(* FB_CylinderDiag	- number of control signals控制信号数量:
							one direction is controllable一个方向是可控的
					- type of feedback signal反馈信号的类型:
							feedback in base and work position基准和工作位置的反馈
					- with position diagnosis带位置诊断				*)
					
FUNCTION_BLOCK FB_CylinderDiag EXTENDS FB_Cylinder
VAR_INPUT
	tTimeOut 	 		: TIME;						// Time for watchdog that monitores if cylinder reaches base/work position监视气缸是否到达基准/工作位置的看门狗的时间
END_VAR
VAR_OUTPUT
	bError				: BOOL;						// Error signal (diagnosed from position watchdog)错误信号（由位置看门狗诊断）
	sErrorMsg			: STRING;					// Error message错误消息
END_VAR
VAR
	fbTriggerError		: R_TRIG;					// Trigger to recognize rising edge of error识别错误上升沿的触发器
	bErrorMove			: BOOL;						// Move error移动错误
	fbTimerWatchDog		: TON;						// Watchdog timer for monitoring if cylinder reaches base/work position看门狗计时器，用于监测气缸是否到达基准/工作位置
END_VAR

// =========================================================
;
// =========================================================

METHOD PROTECTED Diag
VAR_INPUT
END_VAR
// =========================================================
// Timer starts when cylinder is not in base and work position当气缸不在基准和工作位置时，计时器启动
	
	IF NOT bAtBasePos AND NOT bAtWorkPos THEN
		fbTimerWatchDog(IN := TRUE,
						PT := tTimeOut);
	ELSE
		fbTimerWatchDog(IN := FALSE,
						PT := tTimeOut);
	END_IF

// =========================================================
// Error if cylinder does not reach base or work position气缸未到达基准或工作位置时报错
	
	fbTriggerError(CLK := fbTimerWatchDog.Q);
	
	bError := fbTimerWatchDog.Q;
	
	IF fbTriggerError.Q THEN
		bErrorMove := bMoveToWork;
	END_IF
	
	IF bError THEN
		IF bErrorMove = bMoveToWork THEN
			IF bMoveToWork THEN
				sErrorMsg := 'Work position not reached';
			ELSE
				sErrorMsg := 'Base position not reached';
			END_IF
		ELSE
			bError := FALSE;
			sErrorMsg := '';
		END_IF
	ELSE
		sErrorMsg := '';
	END_IF

// =========================================================
END_METHOD

METHOD Reset
VAR_INPUT
END_VAR
// =========================================================

// Calling method Reset of base class FB_Cylinder via 'SUPER^.'通过'SUPER^'调用FB_Cylinder的方法Reset
SUPER^.Reset();		

// Reset error重置错误
bError 		:= FALSE;
sErrorMsg 	:= '';

// =========================================================
END_METHOD

METHOD PROTECTED StateMachine
VAR_INPUT
	bBasePosReq		: BOOL;
	bWorkPosReq		: BOOL;
END_VAR
// =========================================================

IF NOT bError THEN
	// Calling method StateMachine of base class FB_Cylinder via 'SUPER^.'通过'SUPER^'调用FB_Cylinder的方法StateMachine
	SUPER^.StateMachine(bBasePosReq := bBasePosReq,
						bWorkPosReq	:= bWorkPosReq );
	
	// Diagnosis诊断
	Diag();
END_IF

// =========================================================
END_METHOD

END_FUNCTION_BLOCK
